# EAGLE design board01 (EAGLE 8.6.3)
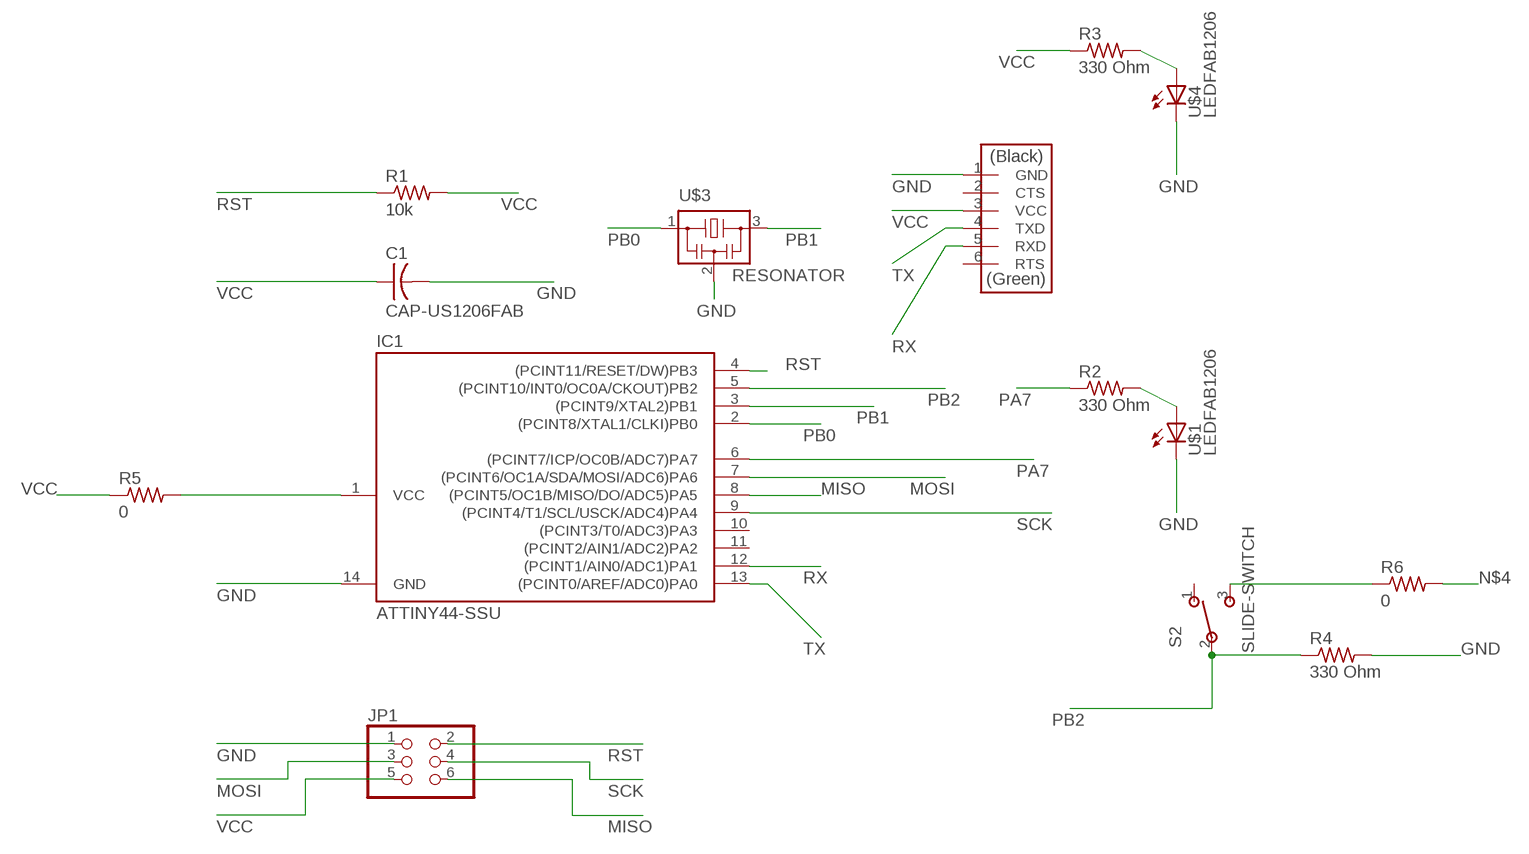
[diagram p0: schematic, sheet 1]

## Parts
C1  CAP-US1206FAB  [C1206FAB]
IC1  ATTINY44-SSU  [SOIC14]
JP1  PINHD-2X3-SMD  [2X03SMD]
R1  10k  RES-US1206FAB  [R1206FAB]
R2  330 Ohm  RES-US1206FAB  [R1206FAB]
R3  330 Ohm  RES-US1206FAB  [R1206FAB]
R4  330 Ohm  RES-US1206FAB  [R1206FAB]
R5  0  RES-US1206FAB  [R1206FAB]
R6  0  RES-US1206FAB  [R1206FAB]
S2  SLIDE-SWITCH  [AYZ0102AGRLC]
U$1  LEDFAB1206  [LED1206FAB]
U$2  FTDI-SMD-HEADER  [1X06SMD]
U$3  RESONATOR  [EFOBM]
U$4  LEDFAB1206  [LED1206FAB]

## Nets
GND: C1.2 IC1.14(GND) JP1.1 R4.2 U$1.2(C) U$2.1(GND) U$3.2 U$4.2(C)
MISO: IC1.8((PCINT5/OC1B/MISO/DO/ADC5)PA5) JP1.6
MOSI: IC1.7((PCINT6/OC1A/SDA/MOSI/ADC6)PA6) JP1.3
N$1: R2.2 U$1.1(A)
N$2: R6.1 S2.3
N$3: R3.2 U$4.1(A)
N$4: IC1.1(VCC) R5.2 R6.2
PA7: IC1.6((PCINT7/ICP/OC0B/ADC7)PA7) R2.1
PB0: IC1.2((PCINT8/XTAL1/CLKI)PB0) U$3.1
PB1: IC1.3((PCINT9/XTAL2)PB1) U$3.3
PB2: IC1.5((PCINT10/INT0/OC0A/CKOUT)PB2) R4.1 S2.2
RST: IC1.4((PCINT11/RESET/DW)PB3) JP1.2 R1.1
RX: IC1.12((PCINT1/AIN0/ADC1)PA1) U$2.5(RXD)
SCK: IC1.9((PCINT4/T1/SCL/USCK/ADC4)PA4) JP1.4
TX: IC1.13((PCINT0/AREF/ADC0)PA0) U$2.4(TXD)
VCC: C1.1 JP1.5 R1.2 R3.1 R5.1 U$2.3(VCC)
Unconnected: IC1.10((PCINT3/T0/ADC3)PA3) IC1.11((PCINT2/AIN1/ADC2)PA2) S2.1 U$2.2(CTS) U$2.6(RTS)

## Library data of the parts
C1 = fab:CAP-US
IC1 = fab:ATTINY44
JP1 = fab:PINHD-2X3-SMD: PIN HEADER
R1-R6 = fab:RES-US: Resistor (US Symbol)
S2 = fab:SLIDE-SWITCH: SMD slide-switch AYZ0102AGRLC as found in the fablab inventory. Includes the mounting holes. Made by Zaerc.
U$1 U$4 = fab:LED: LED
U$2 = fab:FTDI-SMD-HEADER
U$3 = fab:RESONATOR

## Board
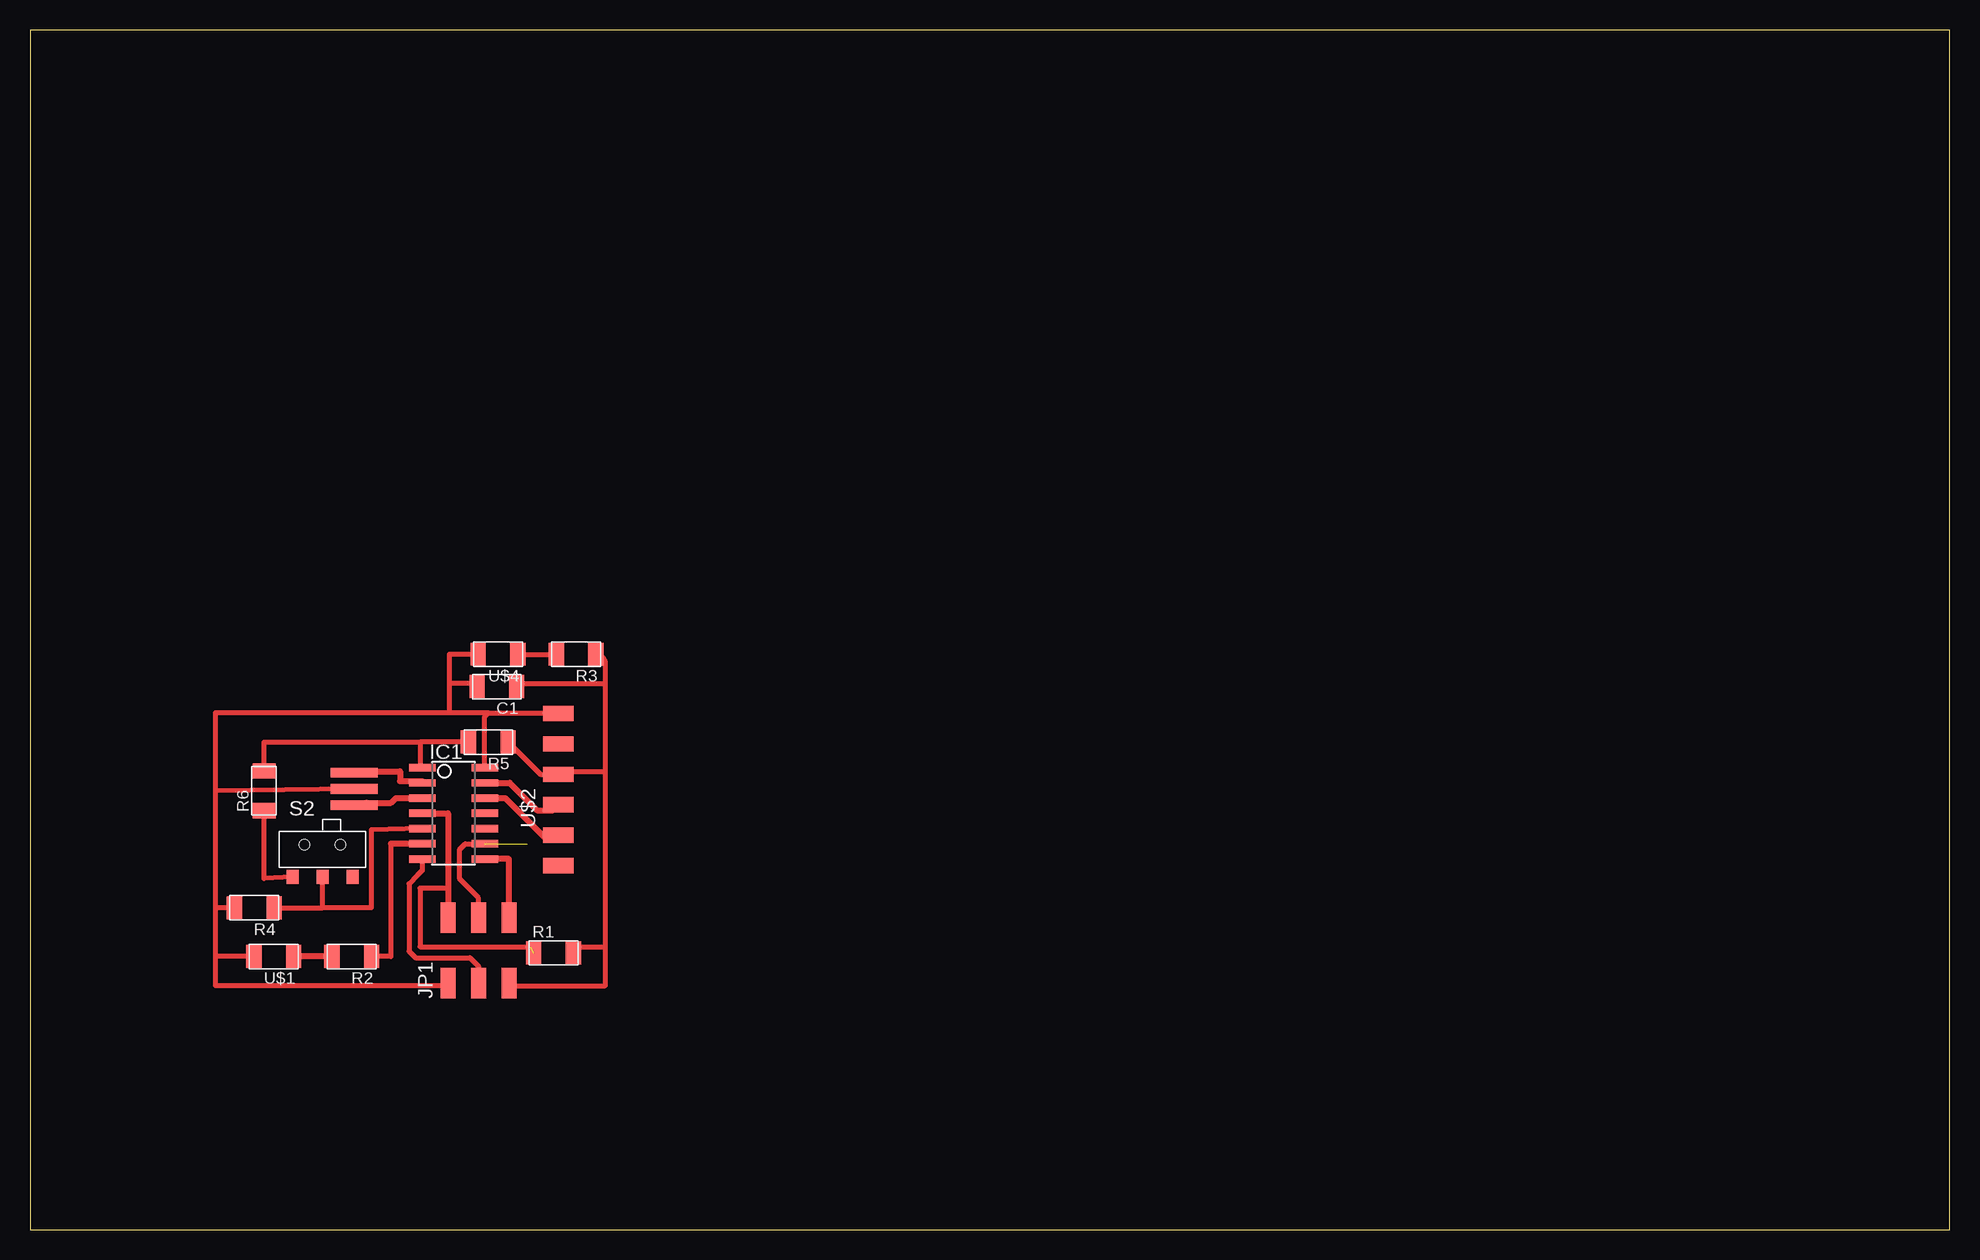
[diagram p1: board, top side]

Size 160 x 100 mm. Coordinates in mm from the lower left corner, seen from the top.
Outline: 0,0 160,0 160,100 0,100 0,0
Copper layers (1*16): Top 0.035mm / dielectric 1.5mm / Bottom 0.035mm
Design rules "default *": minimum track width 6mil, minimum drill 0.35mm, track to track 20mil, track to pad 20mil, pad to pad 20mil, via to via 20mil, smd to smd 20mil, copper to edge 40mil, drill to drill 6mil, minimum pad ring 10mil, minimum via ring 8mil, stop-mask expansion 4mil, vias tented up to drill 0mil, thermal gap 10mil

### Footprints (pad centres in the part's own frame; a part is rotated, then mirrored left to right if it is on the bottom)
C1206FAB = smd 1.27 x 1.905: 1 -1.651,0; 2 1.651,0
SOIC14 = smd 0.61 x 2.21: 1 -3.81,-2.603; 2 -2.54,-2.603; 3 -1.27,-2.603; 4 0,-2.603; 5 1.27,-2.603; 6 2.54,-2.603; 7 3.81,-2.603; 8 3.81,2.603; 9 2.54,2.603; 10 1.27,2.603; 11 0,2.603; 12 -1.27,2.603; 13 -2.54,2.603; 14 -3.81,2.603
2X03SMD = smd 2.54 x 1.27: 1 -2.54,2.54; 2 2.92,2.54; 3 -2.54,0; 4 2.92,0; 5 -2.54,-2.54; 6 2.92,-2.54
R1206FAB = smd 1.27 x 1.905: 1 -1.651,0; 2 1.651,0
AYZ0102AGRLC = smd 1 x 1.2: 1 2.5,-2.3; 2 0,-2.3; 3 -2.5,-2.3 | hole 0.85: -1.5,0.4; 1.5,0.4
LED1206FAB = smd 1.27 x 1.905: 1 -1.651,0; 2 1.651,0
1X06SMD = smd 2.54 x 1.27: 1 0,6.35; 2 0,3.81; 3 0,1.27; 4 0,-1.27; 5 0,-3.81; 6 0,-6.35
EFOBM = smd 0.8 x 3.9: 1 -1.35,0; 2 0,0; 3 1.35,0

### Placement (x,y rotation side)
C1  38.91,45.26 180 top
IC1  35.31,34.7 270 top
JP1  37.39,23.06 90 top
R1  43.64,23.06 0 top
R2  26.82,22.76 180 top
R3  45.52,47.96 180 top
R4  18.69,26.82 180 top
R5  38.2,40.64 180 top
R6  19.51,36.58 90 top
S2  24.38,31.7 0 top
U$1  20.32,22.76 180 top
U$2  44.04,36.68 0 top
U$3  27.03,36.73 270 top
U$4  39.01,47.96 180 top

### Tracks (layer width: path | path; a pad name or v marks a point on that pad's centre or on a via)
GND
  Top 0.406: R4.2 15.44,26.82 | IC1.14 37.91,42.79 38.2,43.08 | 38.2,43.08 43.99,43.08 | 27.69,36.58 arc90 U$3.2 15.44,36.58 | 38.2,43.08 34.95,43.08 | JP1.1 arc-90 34.65,20.32 15.44,20.32 15.44,22.76 | 15.44,26.82 15.44,22.76 | U$1.2 15.44,22.76 | U$4.2 34.95,47.95 34.95,45.52 | 34.95,45.52 34.95,43.08 | C1.2 arc90 37.01,45.52 34.95,45.52 | 34.95,43.08 15.44,43.08 15.44,36.58 | 15.44,36.58 15.44,26.82
  Top 0.508: 43.08,43.08 43.99,43.08 U$2.1
MISO
  Top 0.508: JP1.6 39.93,30.89 IC1.8
MOSI
  Top 0.406: IC1.7 32.7,29.93 32.27,29.5 31.6,28.83 31.6,23.19 32.13,22.66 36.68,22.66 37.39,21.95 JP1.3
N$1
  Top 0.508: R2.2 U$1.1
N$2
  Top 0.406: S2.3 19.51,29.26 R6.1
N$3
  Top 0.406: U$4.1 R3.2
N$4
  Top 0.406: R5.2 32.51,40.64 | 32.51,40.64 32.51,38.51 IC1.1 | R6.2 19.51,40.64 32.51,40.64
PA7
  Top 0.406: 30.07,32.16 30.07,22.76 R2.1
  Top 0.508: IC1.6 30.07,32.16
PB0
  Top 0.508: U$3.1 27.96,38.2 30.84,38.2 30.84,37.39 32.7,37.39 IC1.2
PB1
  Top 0.508: IC1.3 30.5,35.97 30.1,35.57 28.03,35.57 U$3.3
PB2
  Top 0.406: 32.6,33.33 IC1.5 28.45,33.33 28.45,26.82 24.38,26.82 | 24.38,26.82 S2.2 | R4.1 24.38,26.82
  Top 0.508: 32.65,33.38 IC1.5
RST  (1 unrouted)
  Top 0.406: 34.85,28.45 32.51,28.45 32.51,23.57 41.68,23.57
  Top 0.508: IC1.4 34.85,34.7 34.85,28.45 JP1.2
RX
  Top 0.508: IC1.12 39.62,35.97 43.08,32.51 43.69,32.51 U$2.5
SCK  (1 unrouted)
  Top 0.406: JP1.4 37.39,27.64 35.81,29.21 35.81,31.7 36.27,32.16 IC1.9
  Top 0.508: JP1.4 37.39,26.01
TX
  Top 0.508: IC1.13 39.98,37.24 42.27,34.95 43.59,34.95 U$2.4
VCC
  Top 0.406: R5.1 42.55,37.95 U$2.3 arc-90 44.3,38.2 47.95,38.2 | JP1.5 arc90 40.13,20.32 47.95,20.32 47.95,23.57 | R3.1 arc-90 47.95,47.17 47.95,45.52 | 47.95,45.52 47.95,38.2 | 47.95,38.2 47.95,23.57 | R1.2 arc-90 45.8,23.57 47.95,23.57 | C1.1 arc-90 40.82,45.52 47.95,45.52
